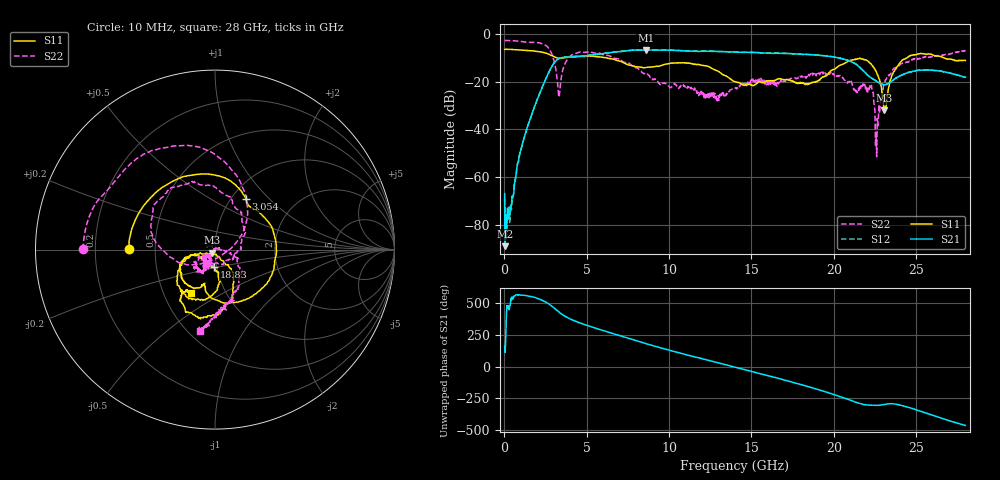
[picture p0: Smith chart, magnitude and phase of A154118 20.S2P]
!  2-Port S-parameters saved by WinCal
! VAR MeasName=S-Parameters (CALIBRATED_DATA) read from VNA (N5230A)
! VAR MeasDate=2015-9-10 14:35:55
! VAR NAME=A154118 20
! VAR FILENAME=A154118 20.S2P
! VAR DATE=2015-9-10 14:35:55
! VAR PHYS_PORTS=1,2
# Hz S DB R 50
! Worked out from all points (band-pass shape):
!   801 points, 10 MHz to 28 GHz, reference 50 ohm
!   highest |S21| = -6.65 dB at 8.582 GHz (marker M1); lowest = -89.1 dB at 44.99 MHz (marker M2)
!   |S21| within 3 dB of the highest: 3.738 GHz to 20.07 GHz (16.33 GHz wide, 137 % of centre)
!   lowest |S11| = -32.0 dB at 23.07 GHz (marker M3), VSWR 1.05, Z = 48.1 - j1.6 ohm
!   |S11| at or under -10 dB: 3.189 GHz to 3.597 GHz (408 MHz wide, 12 % of centre); 6.198 GHz to 24.44 GHz (18.24 GHz wide, 119 % of centre); 26.72 GHz to end of sweep
!   |S22| runs from -51.5 to -2.7 dB; largest |S21 - S12| = 0.0077
!   S11 on the Smith chart (normalised r, x): 10 MHz: 0.35, +0.00; 3.054 GHz: 1.17, +0.74; 18.83 GHz: 0.97, -0.19; 28 GHz: 0.68, -0.36
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1e7  -6.42 179.5  -67.03 160.0  -69.26 -153.6  -2.66 179.8
4.49875e7  -6.38 178.4  -89.09 110.9  -79.09 -112.8  -2.69 178.9
2.549125e8  -6.39 170.3  -77.59 120.6  -77.49 103.7  -2.71 173.7
1.024638e9  -6.72 142.3  -48.05 -156.3  -47.97 -156.2  -3.12 154.9
2.319175e9  -7.64 90.2  -21.89 161.5  -21.87 161.8  -4.12 111.8
3.053912e9  -9.62 58.5  -11.80 97.8  -11.78 97.9  -12.34 42.8
3.333812e9  -10.20 52.5  -10.18 67.6  -10.16 67.6  -25.91 -83.1
4.698325e9  -9.31 -4.4  -9.33 -20.8  -9.31 -20.7  -7.53 140.7
6.692612e9  -10.76 -84.4  -7.55 -103.9  -7.48 -104.1  -10.13 80.0
8.581938e9  -14.03 -107.7  -6.65 -178.7  -6.62 -179.1  -16.71 3.6
9.351662e9  -13.52 -110.5  -6.77 153.1  -6.71 152.7  -20.55 -35.3
1.138094e10  -12.49 -141.7  -7.18 82.2  -7.15 81.6  -22.95 -134.9
1.4005e10  -20.04 -162.0  -7.53 -4.7  -7.51 -5.3  -22.89 -115.0
1.655909e10  -18.94 -122.7  -8.06 -90.2  -7.98 -90.7  -21.94 -127.4
1.869332e10  -20.19 -97.8  -8.67 -167.5  -8.67 -167.9  -16.41 -116.3
1.883328e10  -20.23 -93.9  -8.73 -172.9  -8.70 -173.1  -17.38 -119.1
2.226205e10  -12.44 -150.0  -18.31 55.5  -18.27 54.2  -22.16 -154.0
2.264691e10  -16.93 -165.8  -19.94 53.6  -19.98 53.0  -35.50 47.5
2.306676e10  -32.04 -138.3  -21.26 60.3  -21.24 59.8  -20.99 -11.1
2.334666e10  -22.12 -53.7  -20.67 66.4  -20.62 65.4  -17.18 -20.4
2.471118e10  -8.97 -86.1  -15.81 31.3  -15.82 29.9  -10.84 -69.5
2.8e10  -11.09 -119.3  -18.14 -104.7  -18.18 -105.5  -6.75 -100.6
